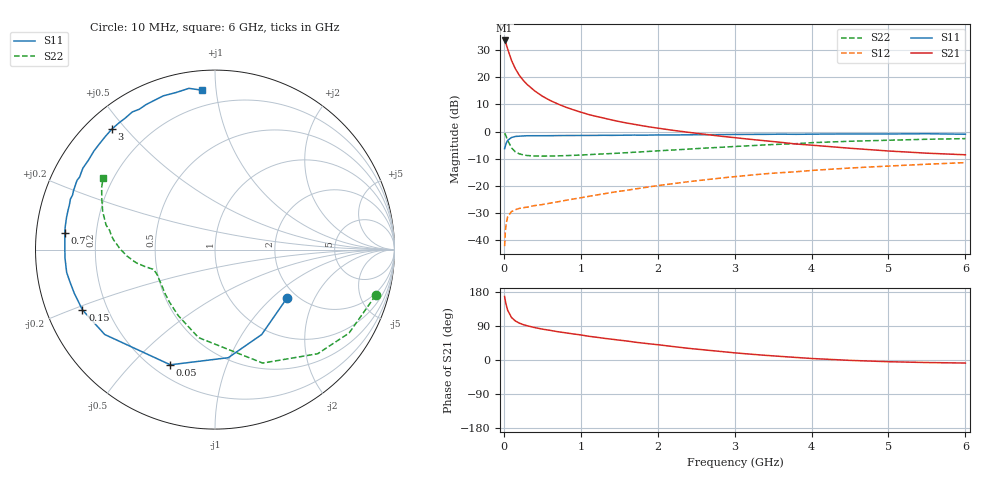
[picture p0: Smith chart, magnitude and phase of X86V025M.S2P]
! SIEMENS Small Signal Semiconductors
! BFP136W
! Si NPN RF Bipolar Junction Transistor in SOT343
! VCE = 6 V  IC = 25 mA
! Common Emitter S-Parameters:  September  1994
# GHz  S  MA  R  50
!  f  S11  S21  S12  S22
! GHz  MAG  ANG  MAG  ANG  MAG  ANG  MAG  ANG
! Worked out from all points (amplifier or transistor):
!   40 points, 10 MHz to 6 GHz, reference 50 ohm
!   highest |S21| = 33.7 dB at 10 MHz (marker M1)
!   |S21| within 3 dB of that: start of sweep to 47.95 MHz
!   unconditionally stable (mu >= 1): 879.8 MHz to 2.817 GHz
!   at 200 MHz: K = 0.37, MSG = 24.6 dB, |S12| = -28.4 dB
!   at 1.5 GHz: K = 1.13, MAG = 10.7 dB, |S12| = -22.1 dB
!   at 6 GHz: K = 0.97, MSG = 1.5 dB, |S12| = -11.5 dB
!   S11 on the Smith chart (normalised r, x): 10 MHz: 1.78, -1.25; 50 MHz: 0.27, -0.65; 150 MHz: 0.11, -0.21; 700 MHz: 0.09, +0.06; 3 GHz: 0.07, +0.46; 6 GHz: 0.11, +0.91
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0.01  0.4834 -33.9  48.29 167.5  0.0076 76.5  0.9306 -15.9
0.02  0.54 -61.2  44.8 155.8  0.0141 67.4  0.8798 -31.9
0.03  0.6068 -83.0  41.51 146.1  0.0198 58.7  0.8149 -45.4
0.05  0.6884 -111.2  33.44 131.1  0.0266 45.7  0.6857 -67.2
0.1  0.7754 -142.4  20.63 112.1  0.0332 32.0  0.4989 -100.6
0.15  0.8113 -155.5  14.47 103.0  0.0359 28.6  0.4209 -119.1
0.2  0.821 -162.8  11.01 97.4  0.0379 27.1  0.3876 -130.8
0.25  0.8287 -167.8  8.922 93.5  0.0391 27.1  0.371 -138.5
0.3  0.8362 -171.3  7.485 90.5  0.0399 28.0  0.3606 -143.9
0.4  0.837 -176.8  5.655 85.6  0.0428 30.1  0.3532 -151.1
0.5  0.8368 179.4  4.512 81.5  0.0447 32.6  0.3512 -155.5
0.6  0.8381 176.6  3.764 78.3  0.0474 35.0  0.3526 -158.1
0.7  0.8417 173.6  3.245 74.7  0.0502 37.8  0.355 -159.7
0.9  0.8451 169.3  2.535 68.8  0.0565 41.6  0.3627 -162.4
1.1  0.8477 164.7  2.068 62.7  0.0632 45.0  0.3738 -163.7
1.5  0.8538 157.4  1.528 52.4  0.0785 49.5  0.3992 -166.2
2.2  0.8633 144.9  1.052 35.5  0.1088 51.0  0.4554 -171.7
3  0.8835 130.7  0.771 18.9  0.1467 47.7  0.5291 179.6
3.2  0.8857 127.4  0.719 15.5  0.1559 46.3  0.5463 177.1
4.5  0.9038 108.6  0.491 -1.0  0.2117 35.9  0.6613 161.2
5.5  0.9102 99.2  0.398 -6.7  0.2487 27.6  0.7197 151.4
6  0.8916 94.8  0.372 -8.0  0.2664 23.2  0.7401 147.3
